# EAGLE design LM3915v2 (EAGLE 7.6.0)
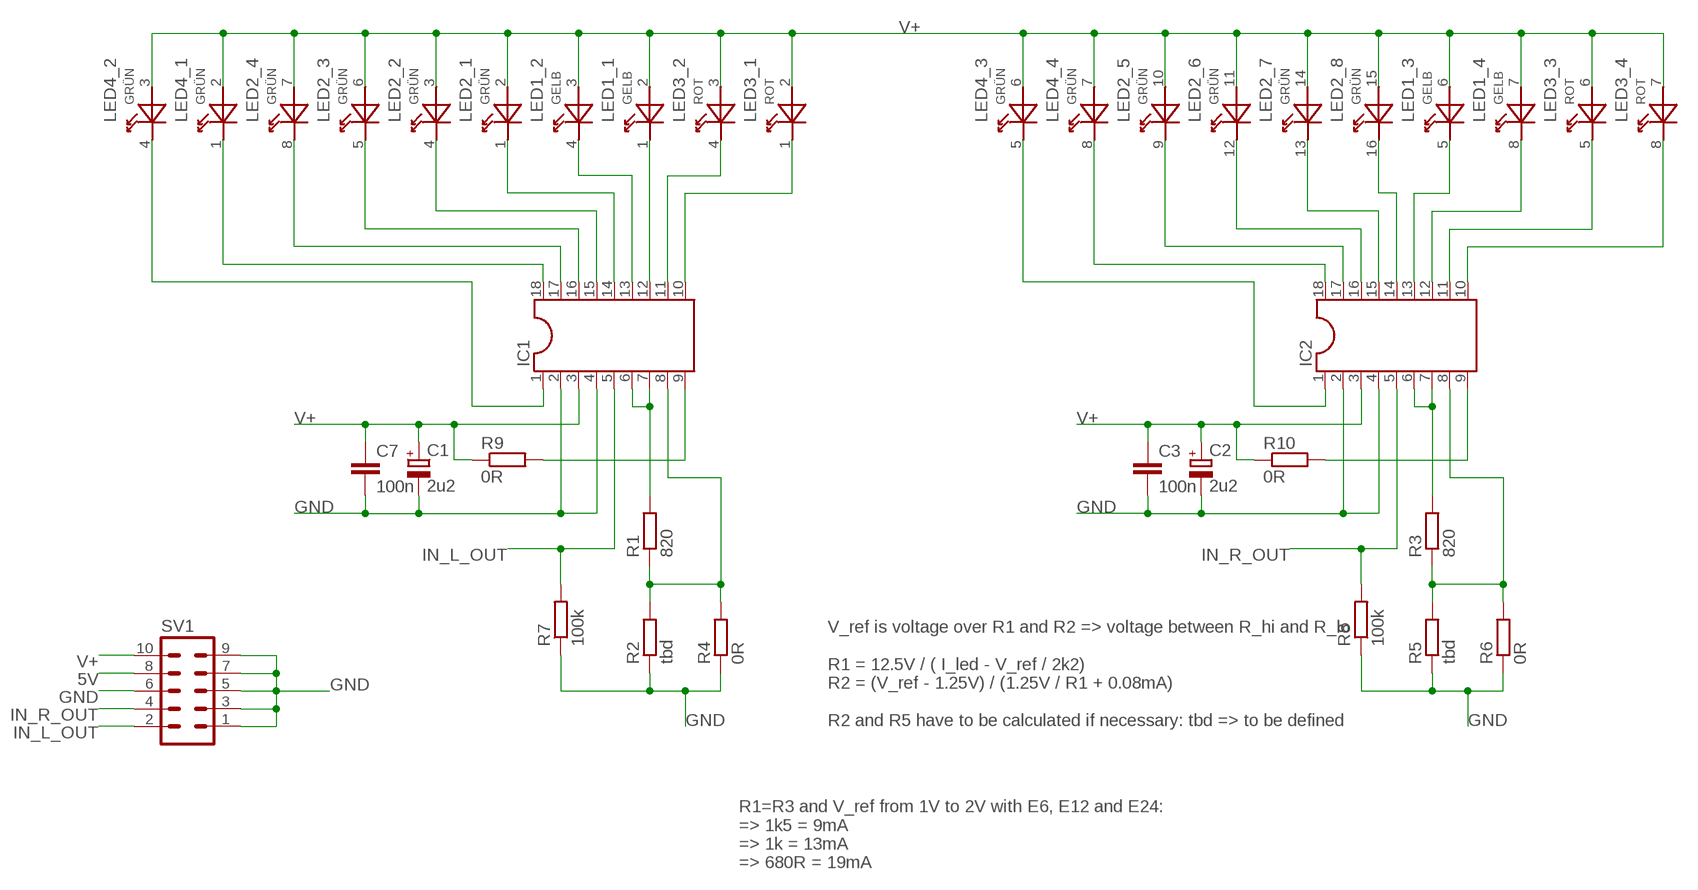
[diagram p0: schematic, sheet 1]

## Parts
C1  2u2  CPOL-EUE2-5  [E2-5]
C2  2u2  CPOL-EUE2-5  [E2-5]
C3  100n  C-EU050-025X075  [C050-025X075]
C7  100n  C-EU050-025X075  [C050-025X075]
IC1  DIL18S  [SOCKET-18]
IC2  DIL18S  [SOCKET-18]
LED1  GELB  KB-27XX-2  [KB-27XX]
LED2  GRÜN  KB-28XX-4  [KB-28XX]
LED3  ROT  KB-27XX-2  [KB-27XX]
LED4  GRÜN  KB-27XX-2  [KB-27XX]
R1  820  R-EU_0309/V  [0309V]
R2  tbd  R-EU_0309/V  [0309V]
R3  820  R-EU_0309/V  [0309V]
R4  0R  R-EU_R0603  [R0603]
R5  tbd  R-EU_0309/V  [0309V]
R6  0R  R-EU_R0603  [R0603]
R7  100k  R-EU_0309/V  [0309V]
R8  100k  R-EU_0309/V  [0309V]
R9  0R  R-EU_R0603  [R0603]
R10  0R  R-EU_R0603  [R0603]
SV1  ML10  [ML10]

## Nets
5V: SV1.8
GND: C1.- C2.- C3.2 C7.2 IC1.2 IC1.4 IC2.2 IC2.4 R2.1 R4.1 R5.1 R6.1 R7.1 R8.1 SV1.1 SV1.3 SV1.5 SV1.6 SV1.7 SV1.9
IN_L_OUT: IC1.5 R7.2 SV1.2
IN_R_OUT: IC2.5 R8.2 SV1.4
N$1: IC1.9 R9.2
N$2: IC1.6 IC1.7 R1.2
N$3: IC1.8 R1.1 R2.2 R4.2
N$4: IC2.6 IC2.7 R3.2
N$5: IC2.9 R10.2
N$6: IC2.8 R3.1 R5.2 R6.2
N$7: IC1.1 LED4.4(_2:P1)
N$8: IC1.18 LED4.1(_1:P1)
N$9: IC1.17 LED2.8(_4:P1)
N$10: IC1.16 LED2.5(_3:P1)
N$11: IC1.15 LED2.4(_2:P1)
N$12: IC1.14 LED2.1(_1:P1)
N$13: IC1.13 LED1.4(_2:P1)
N$14: IC1.12 LED1.1(_1:P1)
N$15: IC1.11 LED3.4(_2:P1)
N$16: IC1.10 LED3.1(_1:P1)
N$18: IC2.18 LED4.8(_4:P1)
N$19: IC2.17 LED2.9(_5:P1)
N$20: IC2.16 LED2.12(_6:P1)
N$21: IC2.15 LED2.13(_7:P1)
N$22: IC2.14 LED2.16(_8:P1)
N$23: IC2.13 LED1.5(_3:P1)
N$24: IC2.12 LED1.8(_4:P1)
N$25: IC2.11 LED3.5(_3:P1)
N$26: IC2.10 LED3.8(_4:P1)
N$27: IC2.1 LED4.5(_3:P1)
V+: C1.+ C2.+ C3.1 C7.1 IC1.3 IC2.3 LED1.2(_1:P2) LED1.3(_2:P2) LED1.6(_3:P2) LED1.7(_4:P2) LED2.2(_1:P2) LED2.3(_2:P2) LED2.6(_3:P2) LED2.7(_4:P2) LED2.10(_5:P2) LED2.11(_6:P2) LED2.14(_7:P2) LED2.15(_8:P2) LED3.2(_1:P2) LED3.3(_2:P2) LED3.6(_3:P2) LED3.7(_4:P2) LED4.2(_1:P2) LED4.3(_2:P2) LED4.6(_3:P2) LED4.7(_4:P2) R9.1 R10.1 SV1.10

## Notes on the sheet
- V_ref is voltage over R1 and R2 => voltage between R_hi and R_lo
  
  R1 = 12.5V / ( I_led - V_ref / 2k2)
  R2 = (V_ref - 1.25V) / (1.25V / R1 + 0.08mA)
  
  R2 and R5 have to be calculated if necessary: tbd => to be defined
- R1=R3 and V_ref from 1V to 2V with E6, E12 and E24:
  => 1k5 = 9mA 
  => 1k = 13mA
  => 680R = 19mA

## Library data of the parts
C1 C2 = rcl:CPOL-EU: POLARIZED CAPACITOR, European symbol
C3 C7 = rcl:C-EU: CAPACITOR, European symbol
IC1 IC2 = ic-package:DIL18: Dual In Line / Socket
LED1 LED3 LED4 = my:KB-27XX-2: FW-LED 10x10 GE reichelt.de
LED2 = my:KB-28XX-4: FW-LED 10X20 GN reichelt.de
R1-R10 = rcl:R-EU_: RESISTOR, European symbol
SV1 = con-ml:ML10: HARTING; OC_FARNELL: unknown; OC_NEWARK: unknown

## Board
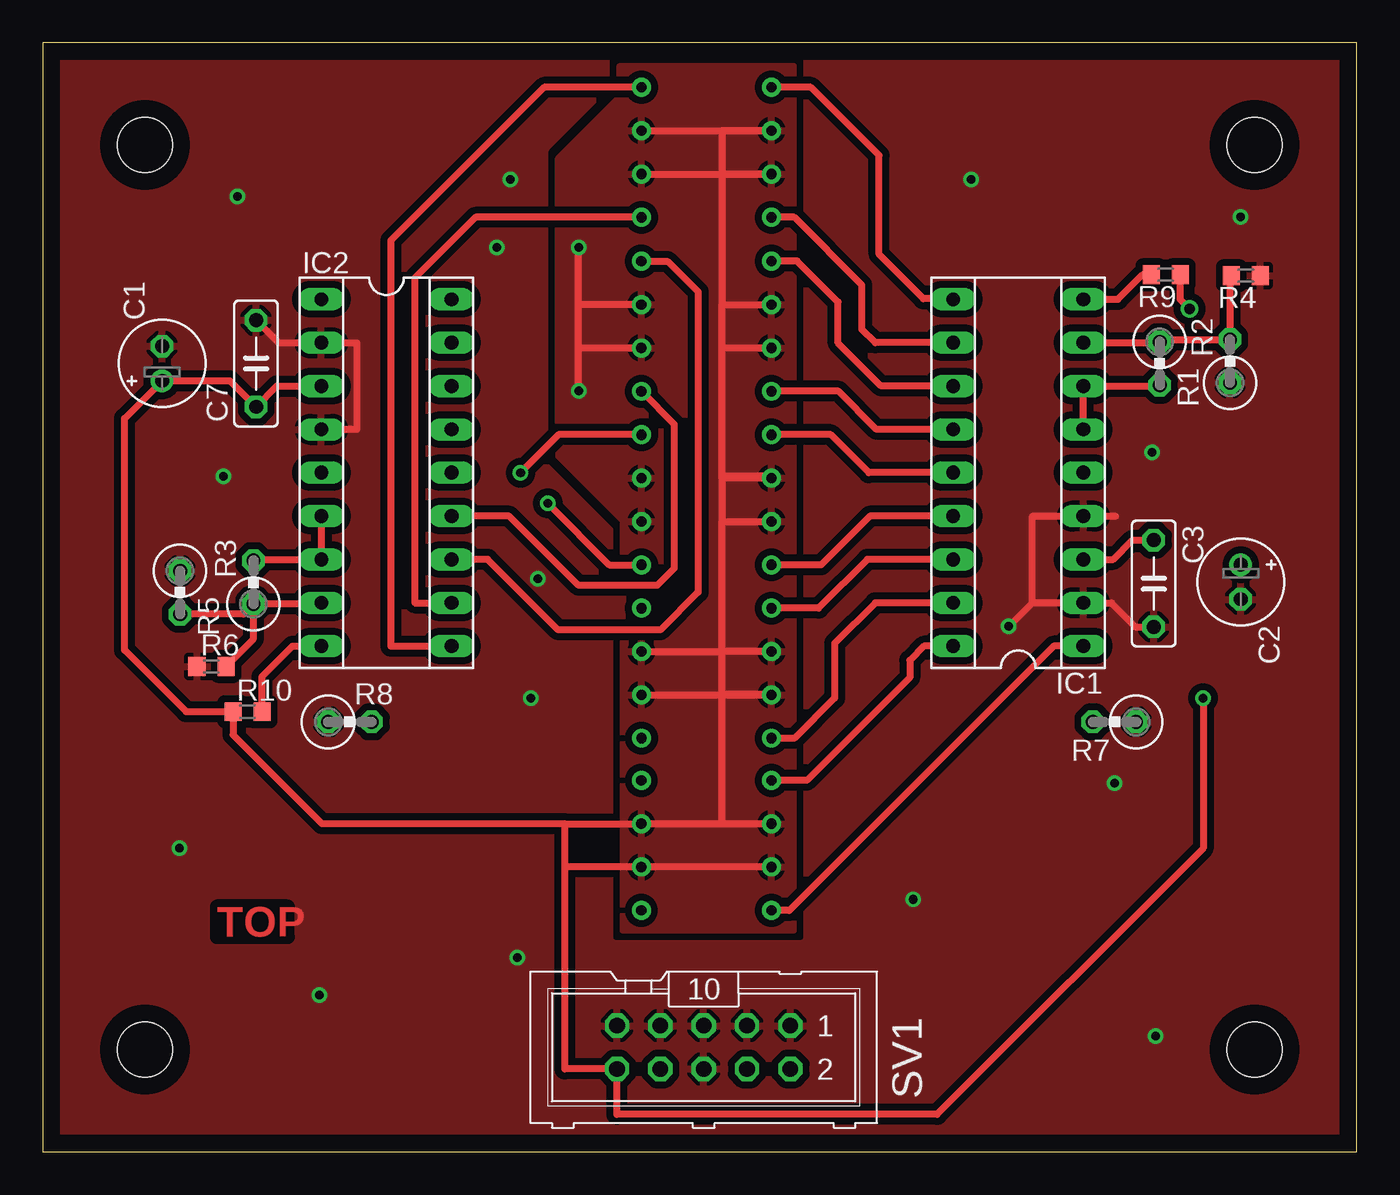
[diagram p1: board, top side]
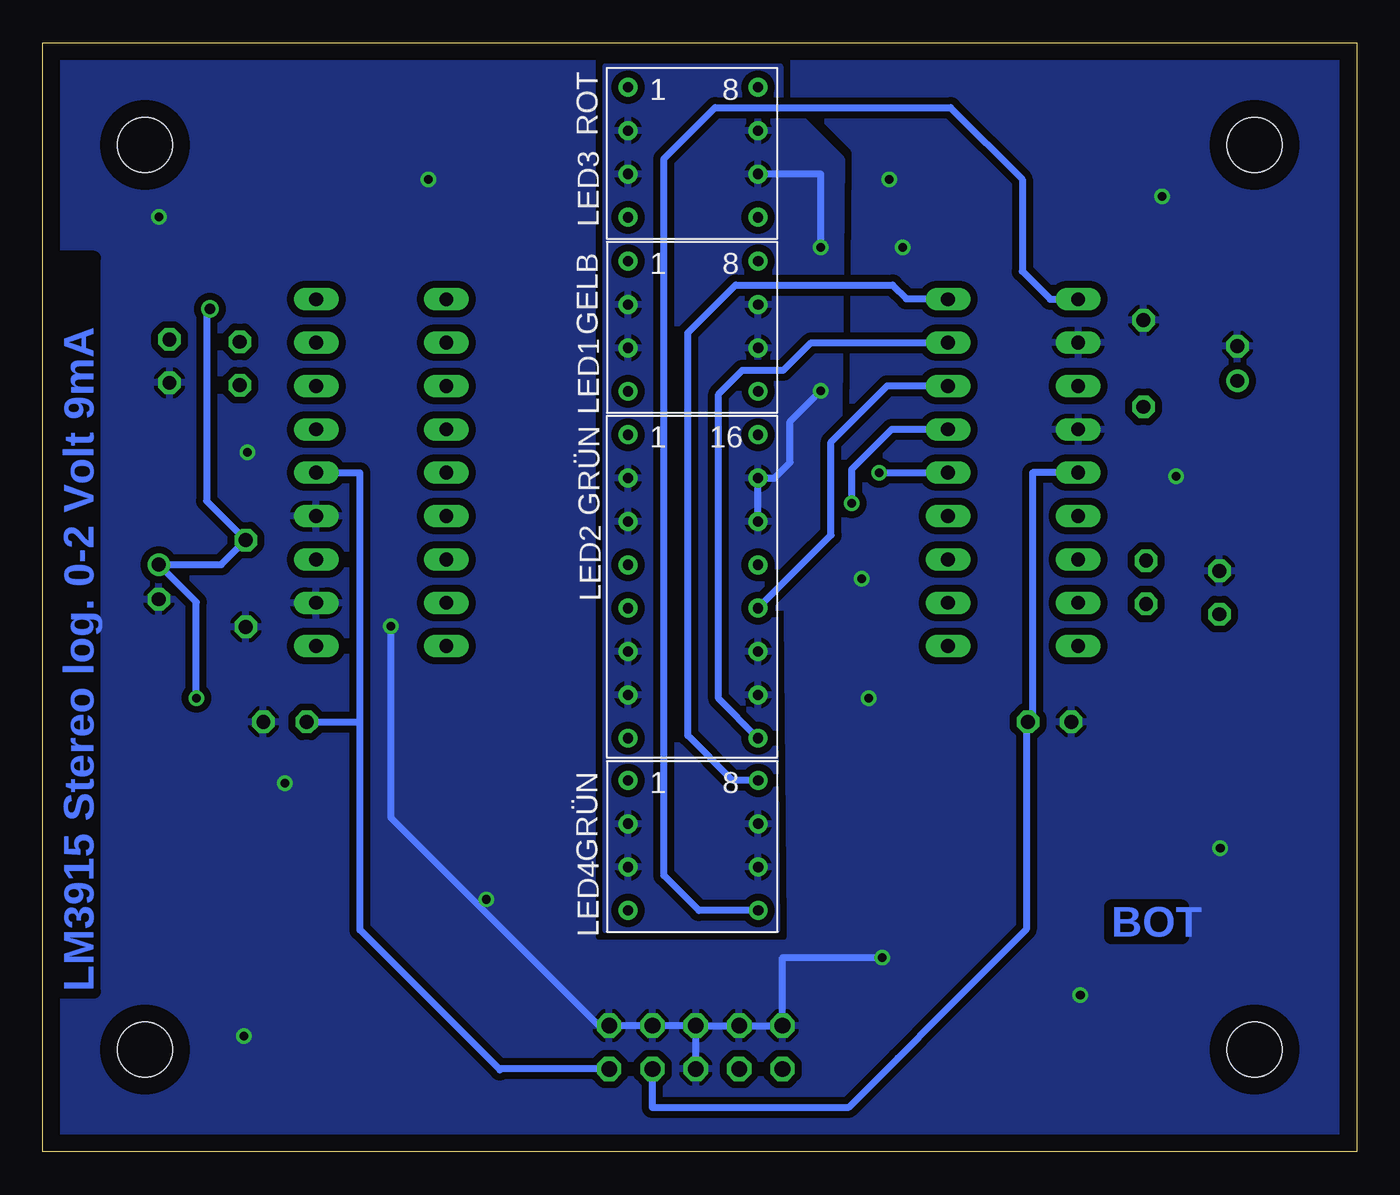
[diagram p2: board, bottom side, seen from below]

Size 77 x 65 mm. Coordinates in mm from the lower left corner, seen from the top.
Outline: 0,0 77,0 77,65 0,65 0,0
Copper layers (1*16): Top 0.035mm / dielectric 1.5mm / Bottom 0.035mm
Design rules "default *": minimum track width 10mil, minimum drill 0.5mm, track to track 8mil, track to pad 8mil, pad to pad 8mil, via to via 8mil, smd to smd 8mil, copper to edge 40mil, drill to drill 8mil, minimum pad ring 10mil, minimum via ring 8mil, stop-mask expansion 4mil, vias tented up to drill 0mil, thermal gap 10mil
Holes 3.2 mm at 6,59 6,6 71,59 71,6

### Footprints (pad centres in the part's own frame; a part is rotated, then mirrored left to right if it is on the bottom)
E2-5 = drill 0.813 pad 1.27: + -1.016,0 | drill 0.813 pad 1.27 octagon: - 1.016,0
C050-025X075 = drill 0.813 octagon: 1 -2.54,0; 2 2.54,0
SOCKET-18 = drill 0.813 long: 1 -10.16,-3.81; 2 -7.62,-3.81; 3 -5.08,-3.81; 4 -2.54,-3.81; 5 0,-3.81; 6 2.54,-3.81; 7 5.08,-3.81; 8 7.62,-3.81; 9 10.16,-3.81; 10 10.16,3.81; 11 7.62,3.81; 12 5.08,3.81; 13 2.54,3.81; 14 0,3.81; 15 -2.54,3.81; 16 -5.08,3.81; 17 -7.62,3.81; 18 -10.16,3.81
KB-27XX = drill 0.6: 1 0,0; 2 0,-2.54; 3 0,-5.08; 4 0,-7.62; 5 7.62,-7.62; 6 7.62,-5.08; 7 7.62,-2.54; 8 7.62,0
KB-28XX = drill 0.6: 1 0,0; 2 0,-2.54; 3 0,-5.08; 4 0,-7.62; 5 0,-10.16; 6 0,-12.7; 7 0,-15.24; 8 0,-17.78; 9 7.62,-17.78; 10 7.62,-15.24; 11 7.62,-12.7; 12 7.62,-10.16; 13 7.62,-7.62; 14 7.62,-5.08; 15 7.62,-2.54; 16 7.62,0
0309V = drill 0.813 octagon: 1 -1.27,0; 2 1.27,0
R0603 = smd 1 x 1.1: 1 -0.85,0; 2 0.85,0
ML10 = drill 0.914 octagon: 1 -5.08,-1.27; 2 -5.08,1.27; 3 -2.54,-1.27; 4 -2.54,1.27; 5 0,-1.27; 6 0,1.27; 7 2.54,-1.27; 8 2.54,1.27; 9 5.08,-1.27; 10 5.08,1.27

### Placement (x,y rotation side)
C1  7,46.2 90 top
C2  70.2,33.4 270 top
C3  65.1,33.31 270 top
C7  12.5,46.2 90 top
IC1  57.16,39.8 90 top
IC2  20.14,39.8 270 top
LED1  42.7,52.19 0 bottom
LED2  42.7,42.02 0 bottom
LED3  42.7,62.38 0 bottom
LED4  42.7,21.77 0 bottom
R1  65.45,46.2 270 top
R2  69.57,46.34 90 top
R3  12.35,33.38 90 top
R4  70.5,51.35 180 top
R5  8.05,32.78 270 top
R6  9.89,28.45 0 top
R7  62.8,25.2 180 top
R8  18,25.2 0 top
R9  65.8,51.4 180 top
R10  12,25.8 0 top
SV1  38.73,6.13 180 top

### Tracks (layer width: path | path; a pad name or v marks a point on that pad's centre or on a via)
GND  (via drill 0.5)
  Top 0.406: 12.5,48.87 C7.2 13.82,47.42 IC2.2 18.4,47.42 18.4,42.34 IC2.4 | 65.17,30.84 C3.2 64.03,30.77 62.62,32.18 IC1.2 58,32.18 | 58,32.18 58,37.26 IC1.4 62.86,37.26 | 58,32.18 56.62,30.8 v56.6,30.8
  Bottom 0.406: SV1.6 SV1.5 | SV1.5 SV1.7 SV1.9 33.65,11.4 v27.8,11.4 | SV1.5 SV1.3 SV1.1 44.4,7.4 56.6,19.6 v56.6,30.8
  other vias: 11.4,56 10.6,39.6 8,17.8 16.2,9.2 51,14.8 62.8,21.6 65.2,6.8 65,41 70.2,54.8 54.4,57 27.4,57 26.6,53 28.6,26.6 29,33.6
  pour Top (isolate 0.406, rank 2): 0.2,64.8 76.8,64.8 76.8,0.2 0.2,0.2
  pour Bottom (isolate 0.406, rank 2): 0.2,64.8 76.8,64.8 76.8,0.2 0.2,0.2
IN_L_OUT
  Bottom 0.406: IC1.5 58.4,39.8 58.4,25.2 | SV1.2 50.2,4.86 50.2,4.8 58.4,13 58.4,25.2 | R7.2 58.4,25.2
IN_R_OUT
  Bottom 0.406: IC2.5 19,39.8 19,25.47 R8.2 19.37,25.1 19.37,13.03 24.4,8 26.9,5.5 29.8,2.6 41.27,2.6 SV1.4
N$1
  Top 0.406: IC1.9 63,49.96 64.44,51.4 R9.2
N$2
  Top 0.406: R1.2 65.4,44.88 IC1.7 IC1.6
N$3
  Top 0.406: IC1.8 65.4,47.42 R1.1 65.59,47.61 R2.2 69.57,51.27 R4.2
N$4
  Top 0.406: R3.2 12.42,34.72 IC2.7 IC2.6
N$5
  Top 0.406: R10.2 12.85,27.85 14.64,29.64 IC2.9
N$6
  Top 0.406: IC2.8 16.26,32.11 R3.1 | R3.1 11.75,31.51 R5.2 | R6.2 12.35,30.06 R3.1
N$7
  Top 0.406: IC1.1 59.24,29.64 43.75,14.15 LED4.4
N$8
  Top 0.406: IC1.18 51.64,29.64 50.8,28.8 50.8,27.8 44.77,21.77 LED4.1
N$9
  Top 0.406: IC1.17 48.78,32.18 46.4,29.8 46.4,26.6 44.04,24.24 LED2.8
N$10
  Top 0.406: IC1.16 48.32,34.72 45.46,31.86 LED2.5
N$11
  Top 0.406: IC1.15 48.46,37.26 45.6,34.4 LED2.4
N$12
  Top 0.406: IC1.14 48.4,39.8 46.18,42.02 LED2.1
N$13
  Top 0.406: IC1.13 48.86,42.34 46.63,44.57 LED1.4
N$14
  Top 0.406: IC1.12 49.12,44.88 46.6,47.4 46.6,49.8 44.2,52.2 LED1.1
N$15
  Top 0.406: IC1.11 48.78,47.42 48,48.2 48,50.8 44.03,54.77 LED3.4
N$16
  Top 0.406: IC1.10 53.31,50 51.6,50 49,52.6 49,58.4 45.02,62.38 LED3.1
N$18
  Bottom 0.406: LED4.8 36.57,21.77 39.2,24.4 39.2,48 36.4,50.8 27.2,50.8 26.4,50 23.99,50 IC2.18
N$19
  Bottom 0.406: LED2.9 37.4,26.56 37.4,44.4 36,45.8 33.6,45.8 31.98,47.42 IC2.17
N$20
  Bottom 0.406: LED2.12 30.8,36.15 30.8,41.6 27.52,44.88 IC2.16
N$21  (via drill 0.5)
  Top 0.406: v29.6,38 33.2,34.4 LED2.13
  Bottom 0.406: IC2.15 27.26,42.34 29.6,40 v29.6,38
N$22  (via drill 0.5)
  Top 0.406: LED2.16 30.22,42.02 v28,39.8
  Bottom 0.406: v28,39.8 IC2.14
N$23
  Top 0.406: LED1.5 37,42.65 37,34.2 36,33.2 31.4,33.2 27.34,37.26 IC2.13
N$24
  Top 0.406: LED1.8 36.61,52.19 38.4,50.4 38.4,32.8 36.2,30.6 30.2,30.6 26.08,34.72 IC2.12
N$25
  Top 0.406: LED3.5 25.36,54.77 21.8,51.2 21.8,32.18 IC2.11
N$26
  Top 0.406: LED3.8 29.39,62.38 20.4,53.4 20.4,29.64 21.8,29.64 22,29.64 IC2.10
N$27
  Bottom 0.406: LED4.5 38.55,14.15 40.6,16.2 40.6,58.2 37.6,61.2 23.8,61.2 19.6,57 19.6,51.6 17.96,49.96 IC2.1
V+  (via drill 0.5, 0.6)
  Top 0.406: IC2.3 13.72,44.88 C7.1 10.98,45.18 C1.+ 4.8,42.98 4.8,29.4 8.4,25.8 R10.1 11.15,24.45 16.37,19.23 30.6,19.23 | 30.6,16.69 30.6,4.86 SV1.10 33.65,2.2 52.4,2.2 68,17.8 v68,26.6 | 30.6,16.69 30.6,19.23 | 30.6,19.23 LED4.7 LED4.2 39.8,19.23 39.8,26.8 | 30.6,16.69 LED4.6 LED4.3 | 65.17,35.92 C3.1 63.85,35.85 62.72,34.72 IC1.3 | LED2.10 LED2.7 42.7,26.8 39.8,26.8 | LED2.11 39.8,29.32 | 39.8,26.8 39.8,29.32 | LED2.6 39.8,29.32 | 39.8,29.32 39.8,36.94 | 39.8,36.94 LED2.3 | 39.8,47.11 39.8,39.6 42.7,39.6 LED2.2 39.8,39.48 39.8,36.94 | 39.8,47.11 39.8,49.65 | 39.8,49.65 LED1.2 | LED1.6 31.4,47.11 | 31.4,47.11 31.4,49.65 | 31.4,49.65 v31.4,53 | LED3.7 LED3.2 39.8,59.84 39.8,57.3 | LED3.6 LED3.3 39.8,57.3 | 39.8,57.3 39.8,49.65 | LED1.7 31.4,49.65 | LED1.3 39.8,47.11 | v31.4,44.6 31.4,47.11 | v67.2,49.4 66.65,49.95 R9.1
  Bottom 0.406: v31.4,53 31.4,57.3 LED3.6 | LED2.14 LED2.15 34.12,39.48 33.2,40.4 33.2,42.8 v31.4,44.6 | v68,26.6 68,32.22 C2.+ 66.53,34.42 C3.1 67.4,38.15 67.4,49.2 v67.2,49.4
  pour Top (isolate 0.406): 33.8,63.6 33.8,61.8 30.2,58.2 30.2,40.8 34,37 34,13 44,13 44,63.6
  pour Bottom (isolate 0.406): 33.8,63.6 33.8,61.8 30.2,58.2 30.4,37.8 34.2,34 34,13 44,13 44,63.6

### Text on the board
Top: TOP
Bottom: BOT | LM3915 Stereo log. 0-2 Volt 9mA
